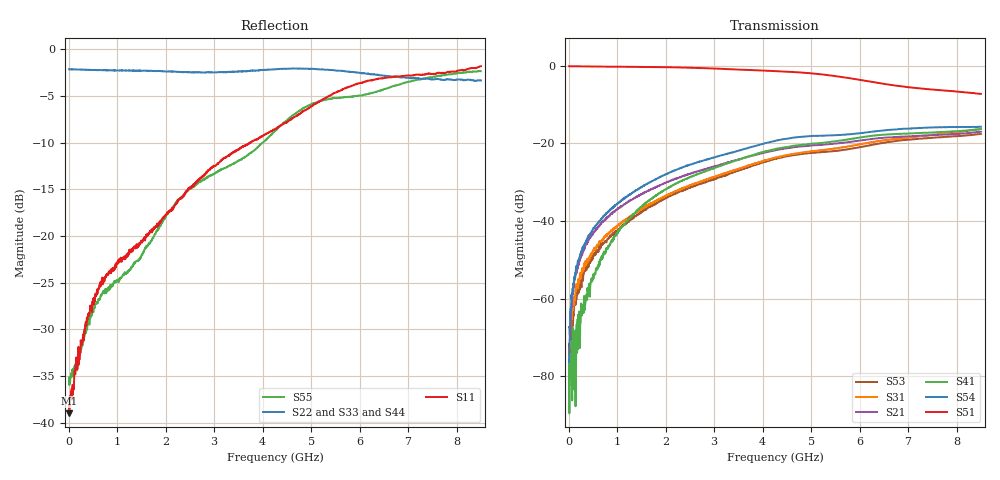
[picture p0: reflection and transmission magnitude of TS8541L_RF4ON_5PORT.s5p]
! Created with skrf (http://scikit-rf.org).
# Hz S RI R 50.0
!freq ReS11 ImS11 ReS12 ImS12 ReS13 ImS13
! ReS14 ImS14 ReS15 ImS15
! ReS21 ImS21 ReS22 ImS22 ReS23 ImS23
! ReS24 ImS24 ReS25 ImS25
! ReS31 ImS31 ReS32 ImS32 ReS33 ImS33
! ReS34 ImS34 ReS35 ImS35
! ReS41 ImS41 ReS42 ImS42 ReS43 ImS43
! ReS44 ImS44 ReS45 ImS45
! ReS51 ImS51 ReS52 ImS52 ReS53 ImS53
! ReS54 ImS54 ReS55 ImS55
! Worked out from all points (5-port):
!   1601 points, 10 MHz to 8.5 GHz, reference 50 ohm
!   strongest paths, dB at 10 MHz, 2.132 GHz, 4.255 GHz, 6.378 GHz, 8.5 GHz:
!     S51: -0.2, -0.4, -1.4, -4.4, -7.3
!     S54: -76.4, -27.2, -19.4, -16.8, -15.7
!     S41: -75.4, -30.9, -21.5, -17.9, -16.3
!     S21: -67.3, -29.4, -21.8, -18.7, -17.0
!     S31: -73.0, -32.7, -23.7, -19.4, -16.3
!     S53: -83.5, -33.2, -24.0, -20.1, -17.6
!   lowest |S11| = -39.0 dB at 15.31 MHz (marker M1), VSWR 1.02, Z = 51.1 - j0.281 ohm
!   |S11| at or under -10 dB: start of sweep to 3.735 GHz; 3.735224 GHz to 3.75203 GHz (16.81 MHz wide, 0.449 % of centre)
